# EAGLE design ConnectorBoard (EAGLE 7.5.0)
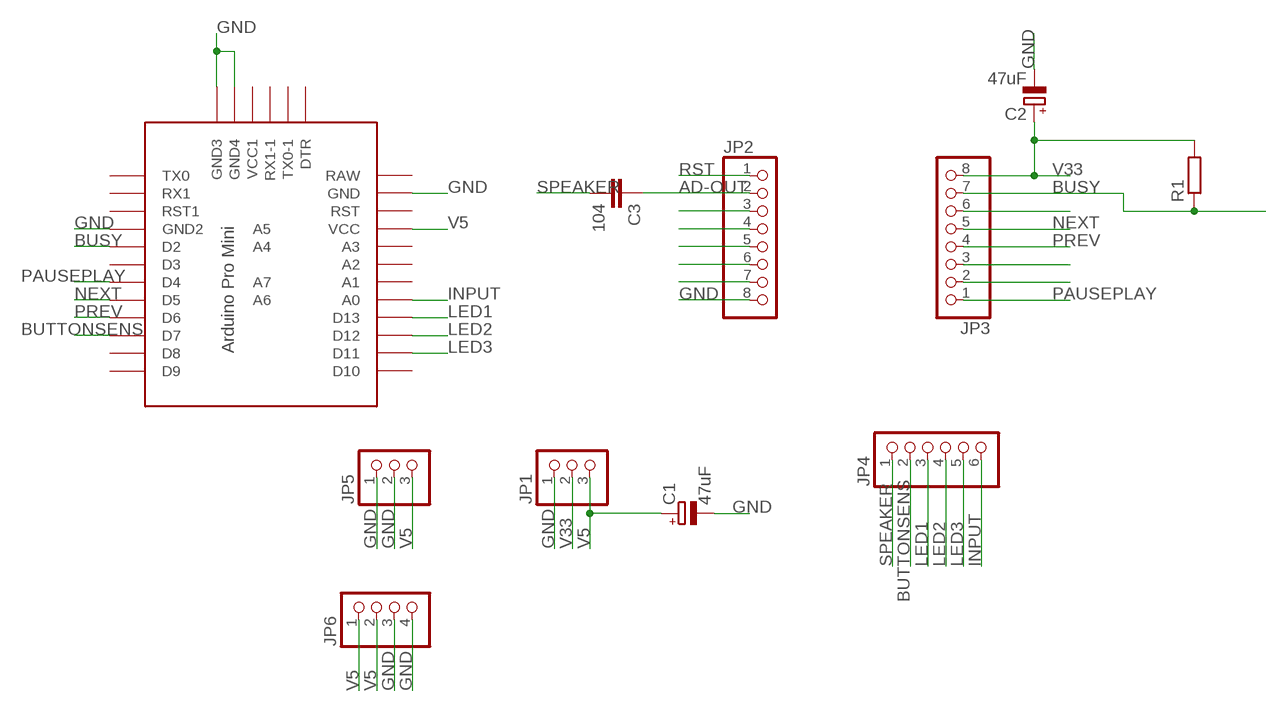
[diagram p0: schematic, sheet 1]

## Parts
C1  47uF  CPOL-EUE5-4  [E5-4]
C2  47uF  CPOL-EUE5-4  [E5-4]
C3  104  C-EU025-024X044  [C025-024X044]
JP1  PINHD-1X3  [1X03]
JP2  PINHD-1X8  [1X08]
JP3  PINHD-1X8  [1X08]
JP4  PINHD-1X6  [1X06]
JP5  PINHD-1X3  [1X03]
JP6  PINHD-1X4  [1X04]
R1  R-EU_0204/2V  [0204V]
U$1  PRO-MINI-2  [PRO-MINI-2]

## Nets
AD-OUT: C3.1 JP2.2
BUSY: JP3.7 R1.1 U$1.D2
BUTTONSENS: JP4.2 U$1.D7
GND: C1.- C2.- JP1.1 JP2.8 JP5.1 JP5.2 JP6.3 JP6.4 U$1.GND U$1.GND1(GND2) U$1.GND2(GND3) U$1.GND3(GND4)
INPUT: JP4.6 U$1.A0
LED1: JP4.3 U$1.D13
LED2: JP4.4 U$1.D12
LED3: JP4.5 U$1.D11
N$3: JP2.3
N$4: JP2.4
N$5: JP2.5
N$6: JP2.6
N$7: JP2.7
N$11: JP3.6
N$14: JP3.3
N$15: JP3.2
NEXT: JP3.5 U$1.D5
PAUSEPLAY: JP3.1 U$1.D4
PREV: JP3.4 U$1.D6
RST: JP2.1
SPEAKER: C3.2 JP4.1
V5: C1.+ JP1.3 JP5.3 JP6.1 JP6.2 U$1.VCC
V33: C2.+ JP1.2 JP3.8 R1.2
Unconnected: U$1.A1 U$1.A2 U$1.A3 U$1.A4 U$1.A5 U$1.A6 U$1.A7 U$1.D3 U$1.D8 U$1.D9 U$1.D10 U$1.DTR U$1.RAW U$1.RST U$1.RST1 U$1.RX1 U$1.RX1-1 U$1.TX0 U$1.TX0-1 U$1.VCC1

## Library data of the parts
C1 C2 = rcl:CPOL-EU: POLARIZED CAPACITOR, European symbol
C3 = rcl:C-EU: CAPACITOR, European symbol
JP1 JP5 = pinhead:PINHD-1X3: PIN HEADER
JP2 JP3 = pinhead:PINHD-1X8: PIN HEADER
JP4 = pinhead:PINHD-1X6: PIN HEADER
JP6 = pinhead:PINHD-1X4: PIN HEADER
R1 = rcl:R-EU_: RESISTOR, European symbol
U$1 = Arduino-clone:PRO-MINI-2: Arduino Pro Mini Layout 2 Sparkfun.com

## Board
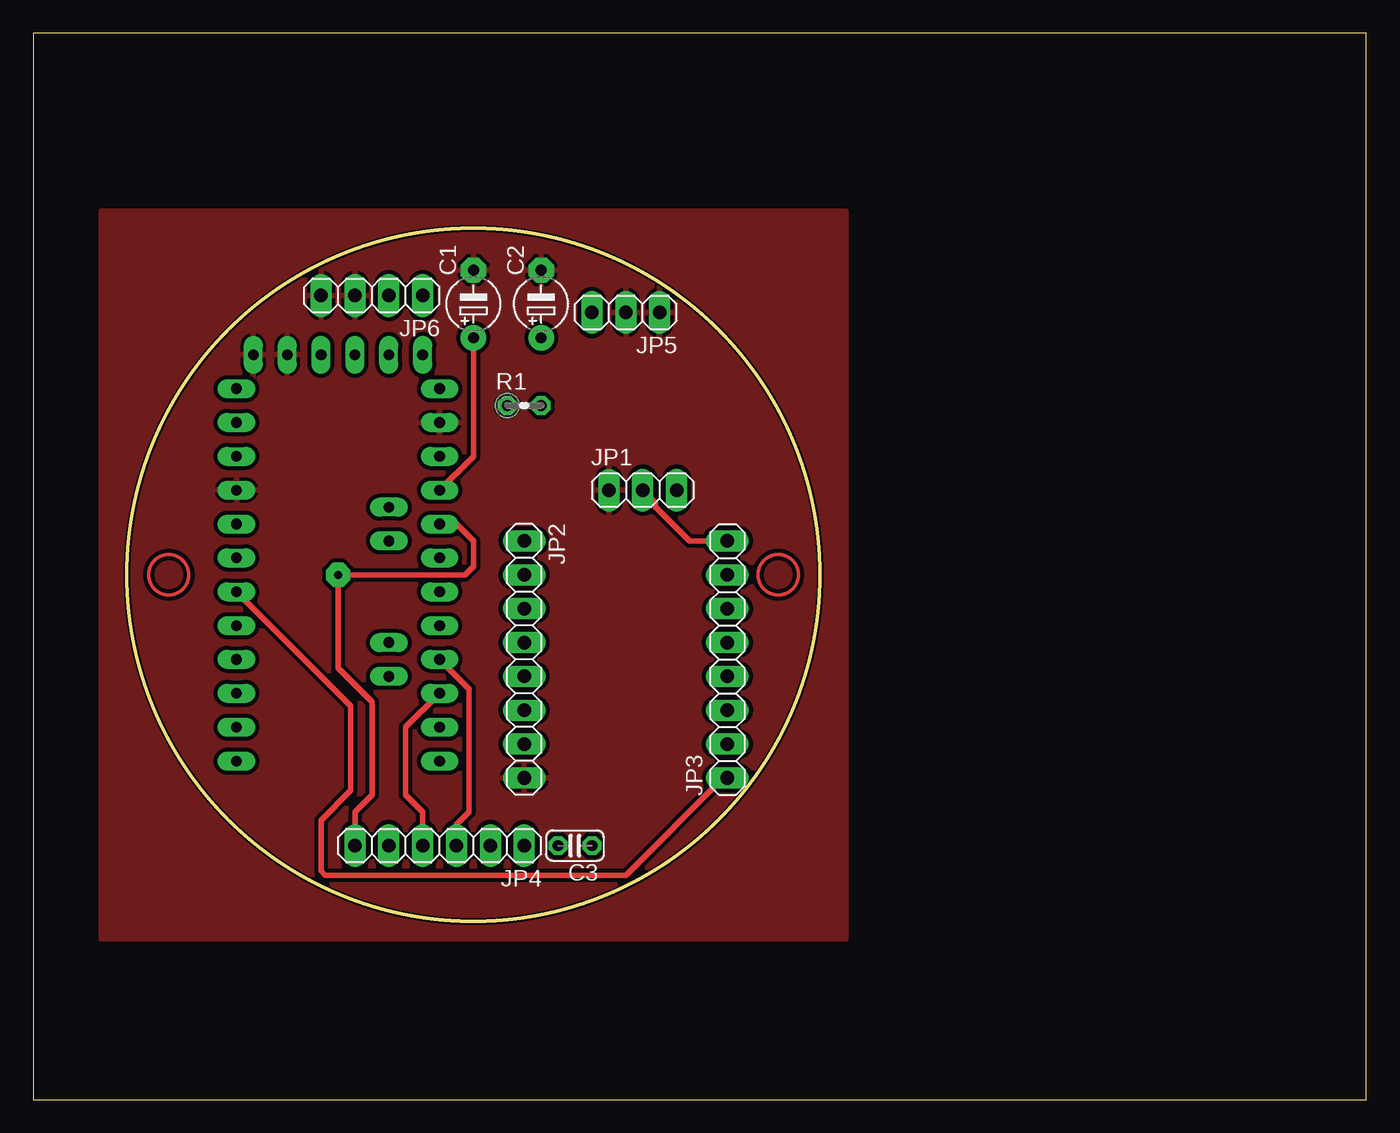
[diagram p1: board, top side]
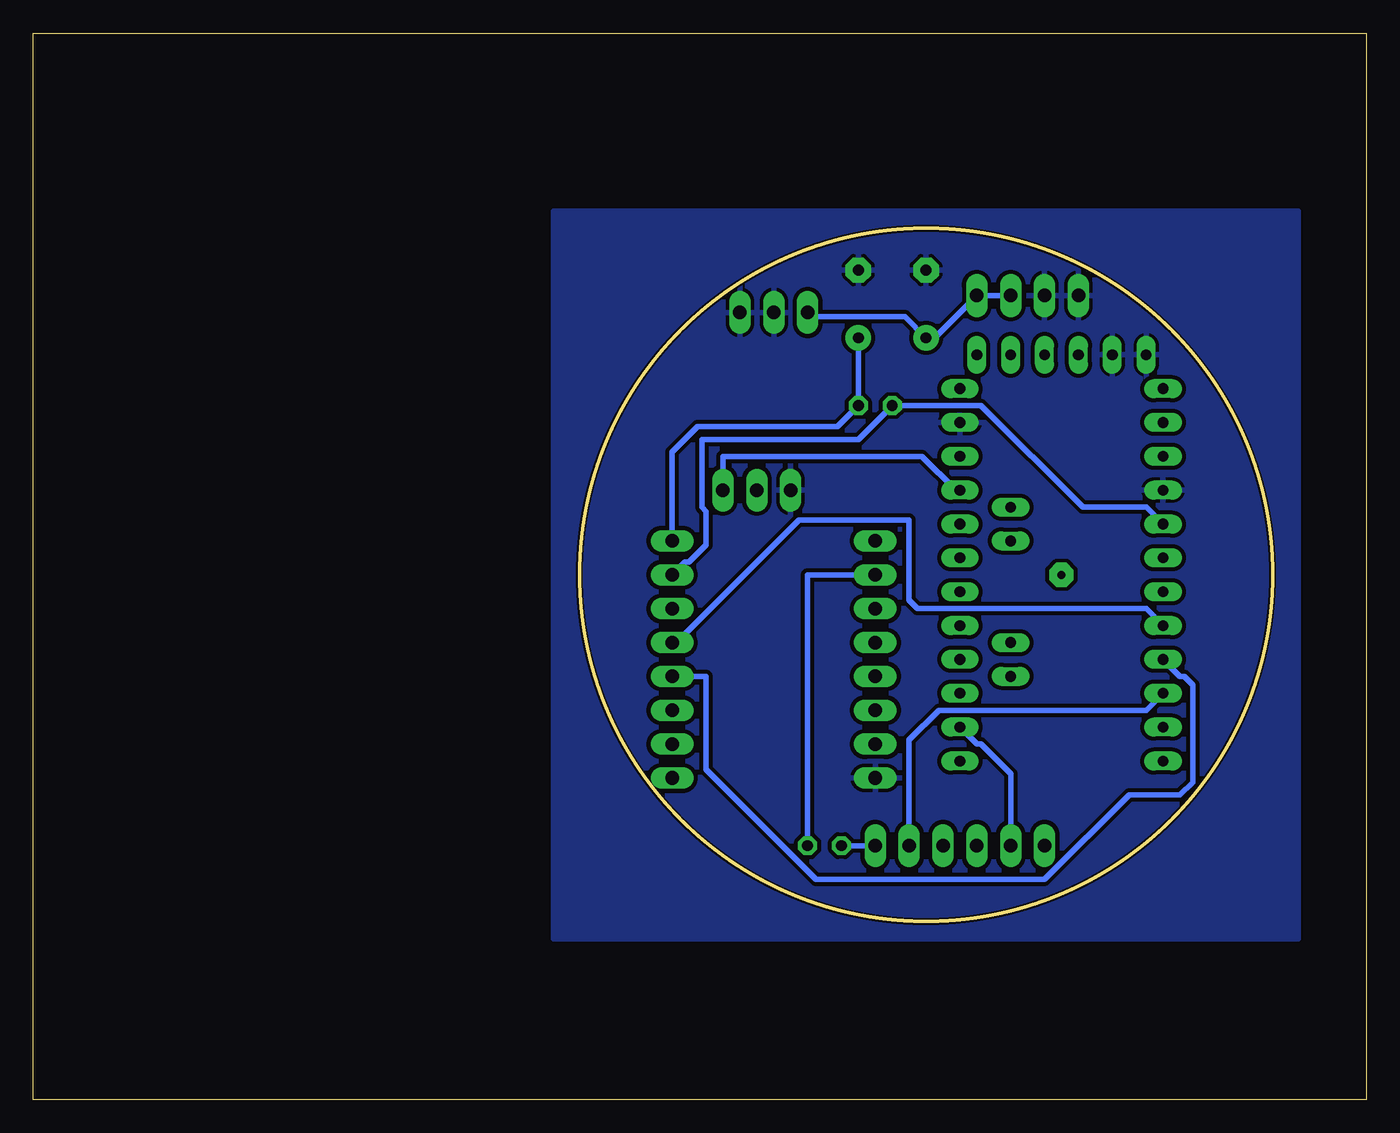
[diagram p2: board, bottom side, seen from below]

Size 100 x 80 mm. Coordinates in mm from the lower left corner, seen from the top.
Outline: 0,0 100,0 100,80 0,80 0,0
Outline: circle at 33.02,39.37 radius 26
Copper layers (1*16): Top 0.035mm / dielectric 1.5mm / Bottom 0.035mm
Design rules "matthias_fein *": minimum track width 16mil, minimum drill 32mil, track to track 12mil, track to pad 12mil, pad to pad 12mil, via to via 12mil, smd to smd 8mil, copper to edge 5mil, drill to drill 8mil, minimum pad ring 12mil, minimum via ring 24mil, stop-mask expansion 4mil, vias tented up to drill 0mil, thermal gap 10mil

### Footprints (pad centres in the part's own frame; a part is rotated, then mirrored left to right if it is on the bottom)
E5-4 = drill 0.813 pad 1.905: + -2.54,0 | drill 0.813 pad 1.905 octagon: - 2.54,0
C025-024X044 = drill 0.813 octagon: 1 -1.27,0; 2 1.27,0
1X03 = drill 1.016 long: 1 -2.54,0; 2 0,0; 3 2.54,0
1X08 = drill 1.016 long: 1 -8.89,0; 2 -6.35,0; 3 -3.81,0; 4 -1.27,0; 5 1.27,0; 6 3.81,0; 7 6.35,0; 8 8.89,0
1X06 = drill 1.016 long: 1 -6.35,0; 2 -3.81,0; 3 -1.27,0; 4 1.27,0; 5 3.81,0; 6 6.35,0
1X04 = drill 1.016 long: 1 -3.81,0; 2 -1.27,0; 3 1.27,0; 4 3.81,0
0204V = drill 0.813 octagon: 1 -1.27,0; 2 1.27,0
PRO-MINI-2 = drill 0.8 long: A0 6.35,2.54; A1 6.35,0; A2 6.35,-2.54; A3 6.35,-5.08; A4 2.54,1.27; A5 2.54,3.81; A6 2.54,-8.89; A7 2.54,-6.35; D2 -8.89,2.54; D3 -8.89,0; D4 -8.89,-2.54; D5 -8.89,-5.08; D6 -8.89,-7.62; D7 -8.89,-10.16; D8 -8.89,-12.7; D9 -8.89,-15.24; D10 6.35,-15.24; D11 6.35,-12.7; D12 6.35,-10.16; D13 6.35,-7.62; DTR 5.08,15.24; GND 6.35,10.16; GND1 -8.89,5.08; GND2 -7.62,15.24; GND3 -5.08,15.24; RAW 6.35,12.7; RST 6.35,7.62; RST1 -8.89,7.62; RX1 -8.89,10.16; RX1-1 0,15.24; TX0 -8.89,12.7; TX0-1 2.54,15.24; VCC 6.35,5.08; VCC1 -2.54,15.24

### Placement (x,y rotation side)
C1  33.02,59.69 90 top
C2  38.1,59.69 90 top
C3  40.64,19.05 180 top
JP1  45.72,45.72 0 top
JP2  36.83,33.02 270 top
JP3  52.07,33.02 90 top
JP4  30.48,19.05 180 top
JP5  44.45,59.05 180 top
JP6  25.4,60.33 180 top
R1  36.83,52.07 0 top
U$1  24.13,40.64 0 top

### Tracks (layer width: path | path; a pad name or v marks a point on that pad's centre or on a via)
AD-OUT
  Bottom 0.406: C3.1 41.91,39.37 JP2.2
BUSY
  Bottom 0.406: U$1.D2 16.51,44.45 21.27,44.45 28.89,52.07 R1.1 38.1,49.53 49.85,49.53 49.85,44.45 49.53,44.13 49.53,41.59 50.8,40.32 51.12,40.32 JP3.7
BUTTONSENS
  Bottom 0.406: U$1.D7 16.51,29.21 32.07,29.21 34.29,26.99 JP4.2
GND
  pour Bottom: 6.99,39.37 arc-90 33.02,65.41 arc-270
  pour Top: 6.99,39.37 arc-90 33.02,65.41 33.66,65.41 arc-90 59.05,40.01 59.05,39.37 arc-90 33.02,13.34 arc-90
INPUT  (via drill 0.6)
  Top 0.406: JP4.6 24.13,21.59 25.4,22.86 25.4,29.84 22.86,32.38 v22.86,39.37 32.38,39.37 33.02,40.01 33.02,41.91 31.75,43.18 U$1.A0
LED1
  Top 0.406: U$1.D13 32.7,30.8 32.7,21.59 31.75,20.64 JP4.3
LED2
  Top 0.406: U$1.D12 27.94,27.94 27.94,22.86 29.21,21.59 JP4.4
LED3
  Bottom 0.406: U$1.D11 29.21,26.67 28.89,26.67 26.67,24.45 JP4.5
N$1
  pour Top: 6.99,39.37 arc-90 33.02,65.41 33.66,65.41 arc-90 59.05,40.01 59.05,39.37 arc-90 33.02,13.34 arc-90
N$2
  pour Bottom: 6.99,39.37 arc-90 33.02,65.41 arc-90 59.05,39.37 arc-90 33.02,13.34 arc-90
N$8
  pour Top: 5.08,66.67 60.96,66.67 60.96,12.06 5.08,12.06
N$9
  pour Bottom: 5.08,66.67 60.96,66.67 60.96,12.06 5.08,12.06
NEXT
  Bottom 0.406: U$1.D5 16.51,36.83 33.66,36.83 34.29,37.47 34.29,43.5 42.55,43.5 51.75,34.29 JP3.5
PAUSEPLAY
  Top 0.406: U$1.D4 23.81,29.53 23.81,23.18 21.59,20.95 21.59,17.14 21.91,16.83 44.45,16.83 51.75,24.13 JP3.1
PREV
  Bottom 0.406: U$1.D6 13.97,31.75 13.65,31.75 13.02,31.11 13.02,23.81 13.97,22.86 17.78,22.86 24.13,16.51 41.27,16.51 49.53,24.77 49.53,31.75 JP3.4
SPEAKER
  Bottom 0.406: JP4.1 C3.2
V5
  Top 0.406: U$1.VCC 33.02,48.26 C1.+
  Bottom 0.406: JP1.3 48.26,48.26 33.34,48.26 30.8,45.72 U$1.VCC | JP5.3 41.59,58.74 34.61,58.74 C1.+ 32.38,57.15 JP6.1 JP6.2
V33
  Top 0.406: JP1.2 46.67,44.77 46.67,44.45 49.21,41.91 JP3.8
  Bottom 0.406: C2.+ R1.2 39.69,50.48 50.16,50.48 52.07,48.58 JP3.8
(copper drawn outside any net)
  shapes: Top circle x2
